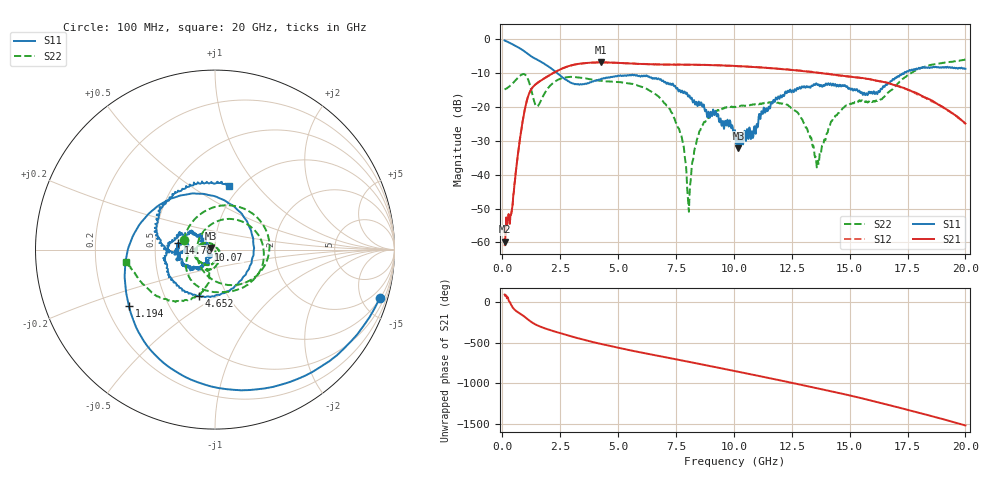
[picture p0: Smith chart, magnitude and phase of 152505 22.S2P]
!  2-Port S-parameters saved by WinCal
! VAR MeasName=S-Parameters (CALIBRATED_DATA) read from VNA (N5230C)
! VAR MeasDate=4/10/2015 9:30:29 AM
! VAR NAME=152505 22
! VAR FILENAME=152505 22.S2P
! VAR DATE=4/10/2015 9:30:29 AM
! VAR PHYS_PORTS=1,2
# Hz S DB R 50
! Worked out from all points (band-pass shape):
!   801 points, 100 MHz to 20 GHz, reference 50 ohm
!   highest |S21| = -6.85 dB at 4.254 GHz (marker M1); lowest = -59.8 dB at 124.9 MHz (marker M2)
!   |S21| within 3 dB of the highest: 2.233 GHz to 13.54 GHz (11.3 GHz wide, 143 % of centre)
!   lowest |S11| = -32.2 dB at 10.2 GHz (marker M3), VSWR 1.05, Z = 47.8 + j0.886 ohm
!   |S11| at or under -10 dB: 2.372 GHz to 17.36 GHz (14.99 GHz wide, 152 % of centre)
!   |S22| runs from -51.0 to -6.0 dB; largest |S21 - S12| = 0.0066
!   S11 on the Smith chart (normalised r, x): 100 MHz: 1.05, -6.80; 1.194 GHz: 0.29, -0.28; 4.652 GHz: 0.74, -0.41; 10.07 GHz: 0.93, -0.00; 14.78 GHz: 0.66, +0.05; 20 GHz: 0.89, +0.73
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1e8  -0.38 -16.4  -59.05 94.0  -61.12 101.1  -14.84 163.0
1.24875e8  -0.46 -20.0  -59.83 78.2  -59.70 83.9  -14.76 158.6
5.72625e8  -1.97 -79.5  -39.87 -103.0  -39.86 -102.8  -12.13 81.9
1.1945e9  -4.83 -146.7  -15.51 127.6  -15.49 127.7  -13.53 -69.7
1.517875e9  -6.10 -175.3  -12.91 73.1  -12.89 73.1  -19.86 165.1
2.214375e9  -9.19 118.3  -9.92 2.1  -9.92 2.0  -12.84 38.3
3.43325e9  -13.38 -25.2  -7.17 -97.9  -7.18 -97.7  -11.43 -44.9
4.254125e9  -11.85 -89.7  -6.85 -155.5  -6.84 -155.5  -12.30 -77.1
4.652125e9  -11.30 -109.7  -6.91 178.7  -6.90 178.8  -12.51 -90.4
6.741625e9  -11.55 172.3  -7.48 56.9  -7.45 56.5  -16.86 -173.7
7.662e9  -14.96 147.5  -7.51 5.7  -7.52 5.8  -27.12 150.1
8.06e9  -16.62 140.3  -7.53 -16.5  -7.52 -16.7  -50.97 -129.8
8.632125e9  -19.85 142.6  -7.58 -49.0  -7.58 -49.2  -25.42 -82.5
1.005e10  -26.87 171.7  -7.90 -130.9  -7.93 -131.0  -20.08 -126.2
1.007488e10  -28.93 -179.5  -7.92 -132.5  -7.96 -132.4  -20.04 -126.3
1.019925e10  -32.17 157.9  -7.96 -139.6  -7.99 -139.3  -19.71 -130.1
1.228875e10  -15.95 -140.7  -8.93 97.5  -8.92 97.3  -19.31 177.7
1.338325e10  -13.83 -163.5  -9.72 30.8  -9.66 30.7  -30.96 112.9
1.365688e10  -13.32 -166.1  -9.93 13.8  -9.87 13.2  -36.84 19.1
1.477625e10  -13.57 169.5  -10.88 -56.4  -10.87 -57.1  -20.00 -91.8
1.669162e10  -13.02 -172.7  -13.00 171.0  -13.04 169.9  -15.60 -100.4
2e10  -8.77 77.9  -24.90 -81.7  -24.99 -80.8  -5.99 -172.0
